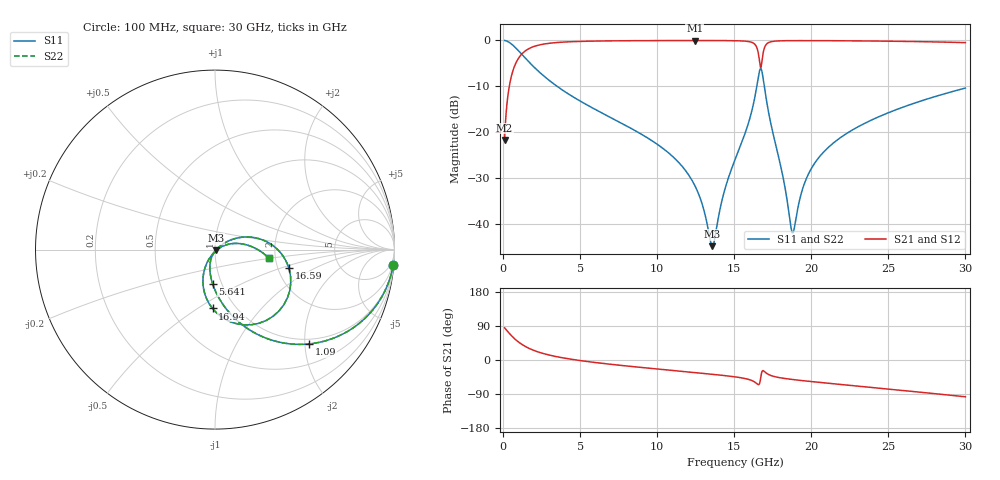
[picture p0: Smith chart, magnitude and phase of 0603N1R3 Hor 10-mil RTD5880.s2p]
# GHz S MA R 50
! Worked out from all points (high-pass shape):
!   3201 points, 100 MHz to 30 GHz, reference 50 ohm
!   highest |S21| = -0.05 dB at 12.44 GHz (marker M1); lowest = -21.7 dB at 100 MHz (marker M2)
!   |S21| within 3 dB of the highest: 1.198 GHz to 16.58 GHz (15.38 GHz wide, 173 % of centre); 16.86 GHz to end of sweep
!   lowest |S11| = -44.8 dB at 13.58 GHz (marker M3), VSWR 1.01, Z = 50.4 - j0.371 ohm
!   |S11| at or under -10 dB: 3.503 GHz to 16.46 GHz (12.96 GHz wide, 130 % of centre); 16.95 GHz to end of sweep
!   |S22| runs from -44.8 to 0.0 dB; largest |S21 - S12| = 0
!   S11 on the Smith chart (normalised r, x): 100 MHz: 1, -23; 1.09 GHz: 0.89, -2.09; 5.641 GHz: 0.91, -0.36; 16.59 GHz: 2.30, -0.57; 16.94 GHz: 0.79, -0.58; 30 GHz: 1.84, -0.19
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0.1  0.9964 -5.0  0.08237 84.9  0.08237 84.9  0.9964 -5.0
0.4830937  0.9285 -23.1  0.3705 66.8  0.3705 66.8  0.9285 -23.1
1.090437  0.7417 -45.1  0.6697 44.8  0.6697 44.8  0.7417 -45.1
2.501344  0.4292 -71.4  0.9014 18.4  0.9014 18.4  0.4292 -71.4
5.089563  0.2143 -91.3  0.974 -2.0  0.974 -2.0  0.2143 -91.3
5.640844  0.1903 -94.1  0.9789 -4.9  0.9789 -4.9  0.1903 -94.1
10.06978  0.07277 -110.8  0.9932 -24.0  0.9932 -24.0  0.07277 -110.8
12.44309  0.02635 -112.3  0.9945 -33.2  0.9945 -33.2  0.02635 -112.3
13.58303  0.005776 -39.5  0.994 -37.7  0.994 -37.7  0.005776 -39.5
14.33987  0.02229 31.3  0.9928 -41.0  0.9928 -41.0  0.02229 31.3
15.05  0.05032 35.3  0.9897 -44.5  0.9897 -44.5  0.05032 35.3
16.29272  0.2211 18.0  0.9204 -57.3  0.9204 -57.3  0.2211 18.0
16.59172  0.424 -14.0  0.6771 -65.0  0.6771 -65.0  0.424 -14.0
16.77859  0.4722 -61.6  0.5584 -33.3  0.5584 -33.3  0.4722 -61.6
16.93744  0.3282 -92.4  0.8058 -29.7  0.8058 -29.7  0.3282 -92.4
17.47938  0.1036 -119.8  0.9723 -42.3  0.9723 -42.3  0.1036 -119.8
18.75947  0.008153 -57.8  0.9916 -51.4  0.9916 -51.4  0.008153 -57.8
19.46025  0.02495 18.5  0.9922 -54.6  0.9922 -54.6  0.02495 18.5
20.03956  0.04132 23.2  0.9919 -57.1  0.9919 -57.1  0.04132 23.2
21.85225  0.08652 21.1  0.989 -64.3  0.989 -64.3  0.08652 21.1
25.01978  0.1636 10.6  0.9785 -76.7  0.9785 -76.7  0.1636 10.6
30  0.3027 -8.8  0.9436 -97.1  0.9436 -97.1  0.3027 -8.8
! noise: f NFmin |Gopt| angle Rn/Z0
0.1  0.00235  0.9895  0.3212  0.05139
3.417  0.004068  0.8115  10.07  0.004467
6.743  0.006815  0.7824  19.23  0.006251
10.06  0.009435  0.769  28.29  0.007831
13.39  0.0127  0.7734  37.2  0.0103
16.7  0.1821  0.9783  46.04  1.616
20.03  0.01717  0.7575  54.63  0.01137
23.35  0.01887  0.7477  62.86  0.01104
26.67  0.02141  0.7492  70.9  0.01153
30  0.02426  0.7539  78.72  0.01206
